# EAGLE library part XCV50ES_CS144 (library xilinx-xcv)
xcv50es_cs144 edit this description Auto generated by make-symbol-device-package-bsdl.ulp Rev. 26 Source: xcv50es_cs144.bsd
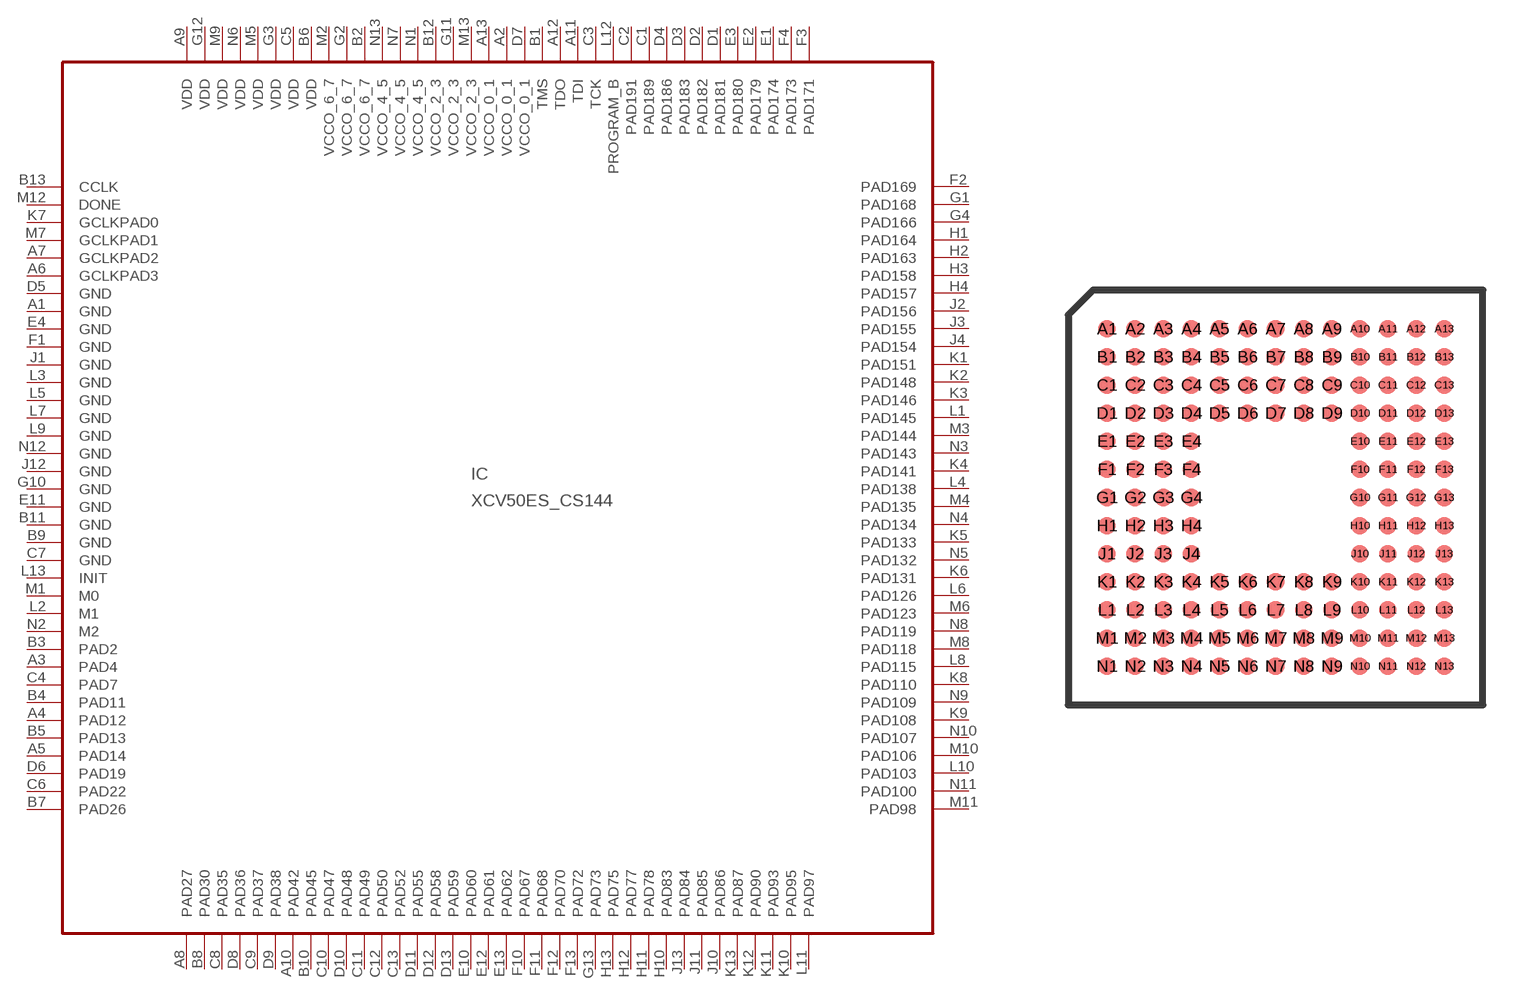
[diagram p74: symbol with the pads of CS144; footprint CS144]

Designator prefix IC

## XCV50ES_CS144 (OC_FARNELL: unknown; OC_NEWARK: unknown)  [CS144]
A1  GND  pwr
A2  VCCO_0_1  pwr
A3  PAD4
A4  PAD12
A5  PAD14
A6  GCLKPAD3  in
A7  GCLKPAD2  in
A8  PAD27
A9  VDD  pwr
A10  PAD42
A11  TDI  in
A12  TDO  out
A13  VCCO_0_1  pwr
B1  TMS  in
B2  VCCO_6_7  pwr
B3  PAD2
B4  PAD11
B5  PAD13
B6  VDD  pwr
B7  PAD26
B8  PAD30
B9  GND  pwr
B10  PAD45
B11  GND  pwr
B12  VCCO_2_3  pwr
B13  CCLK
C1  PAD189
C2  PAD191
C3  TCK  in
C4  PAD7
C5  VDD  pwr
C6  PAD22
C7  GND  pwr
C8  PAD35
C9  PAD37
C10  PAD47
C11  PAD49
C12  PAD50
C13  PAD52
D1  PAD181
D2  PAD182
D3  PAD183
D4  PAD186
D5  GND  pwr
D6  PAD19
D7  VCCO_0_1  pwr
D8  PAD36
D9  PAD38
D10  PAD48
D11  PAD55
D12  PAD58
D13  PAD59
E1  PAD174
E2  PAD179
E3  PAD180
E4  GND  pwr
E10  PAD60
E11  GND  pwr
E12  PAD61
E13  PAD62
F1  GND  pwr
F2  PAD169
F3  PAD171
F4  PAD173
F10  PAD67
F11  PAD68
F12  PAD70
F13  PAD72
G1  PAD168
G2  VCCO_6_7  pwr
G3  VDD  pwr
G4  PAD166
G10  GND  pwr
G11  VCCO_2_3  pwr
G12  VDD  pwr
G13  PAD73
H1  PAD164
H2  PAD163
H3  PAD158
H4  PAD157
H10  PAD83
H11  PAD78
H12  PAD77
H13  PAD75
J1  GND  pwr
J2  PAD156
J3  PAD155
J4  PAD154
J10  PAD86
J11  PAD85
J12  GND  pwr
J13  PAD84
K1  PAD151
K2  PAD148
K3  PAD146
K4  PAD141
K5  PAD133
K6  PAD131
K7  GCLKPAD0  in
K8  PAD110
K9  PAD108
K10  PAD95
K11  PAD93
K12  PAD90
K13  PAD87
L1  PAD145
L2  M1  in
L3  GND  pwr
L4  PAD138
L5  GND  pwr
L6  PAD126
L7  GND  pwr
L8  PAD115
L9  GND  pwr
L10  PAD103
L11  PAD97
L12  PROGRAM_B  in
L13  INIT
M1  M0  in
M2  VCCO_6_7  pwr
M3  PAD144
M4  PAD135
M5  VDD  pwr
M6  PAD123
M7  GCLKPAD1  in
M8  PAD118
M9  VDD  pwr
M10  PAD106
M11  PAD98
M12  DONE
M13  VCCO_2_3  pwr
N1  VCCO_4_5  pwr
N2  M2  in
N3  PAD143
N4  PAD134
N5  PAD132
N6  VDD  pwr
N7  VCCO_4_5  pwr
N8  PAD119
N9  PAD109
N10  PAD107
N11  PAD100
N12  GND  pwr
N13  VCCO_4_5  pwr

## Footprint CS144 (pad centres in mm)
xcv100e_cs144 edit this description Auto generated by make-symbol-device-package-bsdl.ulp Rev. 26 Source: xcv100e_cs144.bsd
smd 0.5 x 0.5: A1 -4.8,4.8; A2 -4,4.8; A3 -3.2,4.8; A4 -2.4,4.8; A5 -1.6,4.8; A6 -0.8,4.8; A7 0,4.8; A8 0.8,4.8; A9 1.6,4.8; A10 2.4,4.8; A11 3.2,4.8; A12 4,4.8; A13 4.8,4.8; B1 -4.8,4; B2 -4,4; B3 -3.2,4; B4 -2.4,4; B5 -1.6,4; B6 -0.8,4; B7 0,4; B8 0.8,4; B9 1.6,4; B10 2.4,4; B11 3.2,4; B12 4,4; B13 4.8,4; C1 -4.8,3.2; C2 -4,3.2; C3 -3.2,3.2; C4 -2.4,3.2; C5 -1.6,3.2; C6 -0.8,3.2; C7 0,3.2; C8 0.8,3.2; C9 1.6,3.2; C10 2.4,3.2; C11 3.2,3.2; C12 4,3.2; C13 4.8,3.2; D1 -4.8,2.4; D2 -4,2.4; D3 -3.2,2.4; D4 -2.4,2.4; D5 -1.6,2.4; D6 -0.8,2.4; D7 0,2.4; D8 0.8,2.4; D9 1.6,2.4; D10 2.4,2.4; D11 3.2,2.4; D12 4,2.4; D13 4.8,2.4; E1 -4.8,1.6; E2 -4,1.6; E3 -3.2,1.6; E4 -2.4,1.6; E10 2.4,1.6; E11 3.2,1.6; E12 4,1.6; E13 4.8,1.6; F1 -4.8,0.8; F2 -4,0.8; F3 -3.2,0.8; F4 -2.4,0.8; F10 2.4,0.8; F11 3.2,0.8; F12 4,0.8; F13 4.8,0.8; G1 -4.8,0; G2 -4,0; G3 -3.2,0; G4 -2.4,0; G10 2.4,0; G11 3.2,0; G12 4,0; G13 4.8,0; H1 -4.8,-0.8; H2 -4,-0.8; H3 -3.2,-0.8; H4 -2.4,-0.8; H10 2.4,-0.8; H11 3.2,-0.8; H12 4,-0.8; H13 4.8,-0.8; J1 -4.8,-1.6; J2 -4,-1.6; J3 -3.2,-1.6; J4 -2.4,-1.6; J10 2.4,-1.6; J11 3.2,-1.6; J12 4,-1.6; J13 4.8,-1.6; K1 -4.8,-2.4; K2 -4,-2.4; K3 -3.2,-2.4; K4 -2.4,-2.4; K5 -1.6,-2.4; K6 -0.8,-2.4; K7 0,-2.4; K8 0.8,-2.4; K9 1.6,-2.4; K10 2.4,-2.4; K11 3.2,-2.4; K12 4,-2.4; K13 4.8,-2.4; L1 -4.8,-3.2; L2 -4,-3.2; L3 -3.2,-3.2; L4 -2.4,-3.2; L5 -1.6,-3.2; L6 -0.8,-3.2; L7 0,-3.2; L8 0.8,-3.2; L9 1.6,-3.2; L10 2.4,-3.2; L11 3.2,-3.2; L12 4,-3.2; L13 4.8,-3.2; M1 -4.8,-4; M2 -4,-4; M3 -3.2,-4; M4 -2.4,-4; M5 -1.6,-4; M6 -0.8,-4; M7 0,-4; M8 0.8,-4; M9 1.6,-4; M10 2.4,-4; M11 3.2,-4; M12 4,-4; M13 4.8,-4; N1 -4.8,-4.8; N2 -4,-4.8; N3 -3.2,-4.8; N4 -2.4,-4.8; N5 -1.6,-4.8; N6 -0.8,-4.8; N7 0,-4.8; N8 0.8,-4.8; N9 1.6,-4.8; N10 2.4,-4.8; N11 3.2,-4.8; N12 4,-4.8; N13 4.8,-4.8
